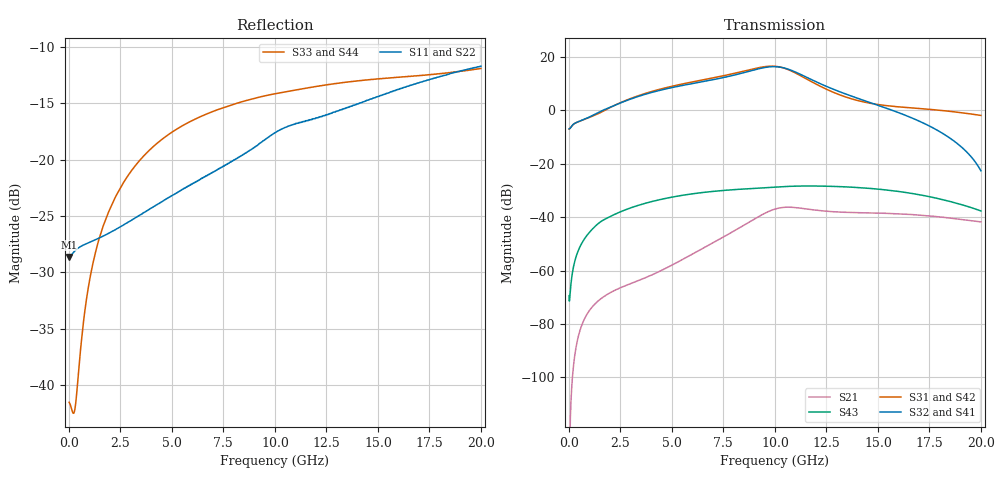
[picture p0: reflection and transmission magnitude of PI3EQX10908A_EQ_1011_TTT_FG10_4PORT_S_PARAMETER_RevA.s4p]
! NPort=4 DATA=2000 NOISE=0 GROUPDELAY=0 COMPLEX_DATAFORMAT=POLAR
! NumOfBlock=1 NumOfParam=0
! .MODEL Smodel S TSTONEFILE=PI3EQX10908A_EQ_1011_TTT_FG10_4PORT_S_PARAMETER_RevA.s4p TYPE=S
!  -- The above .MODEL line can be used for the S element in the netlist.
! The s parameter is extracted from the linear redriver, it is not bi-directional; only s(4,1)s(4,2) and s(3,1)s(3,2)
! should be the insertion loss
!Port definition:
!Port1 = input+
!Port2 = input-
!Port3 = output+
!Port4 = output-
# Hz S MA R  50
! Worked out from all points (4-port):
!   2000 points, 10 MHz to 20 GHz, reference 50 ohm
!   strongest paths, dB at 10 MHz, 5.01 GHz, 10.01 GHz, 15.01 GHz, 20 GHz:
!     S32: -6.9, 8.6, 16.4, 1.9, -22.6
!     S41: -6.9, 8.6, 16.4, 1.9, -22.5
!     S31: -6.9, 9.1, 16.5, 2.2, -1.9
!     S42: -6.9, 9.1, 16.5, 2.2, -1.8
!     S43: -69.4, -32.4, -28.7, -29.5, -37.6
!     S21: -127.2, -57.9, -36.9, -38.4, -41.7
!   lowest |S11| = -28.6 dB at 10 MHz (marker M1), VSWR 1.08, Z = 46.4 - j0.024 ohm
!   |S11| at or under -10 dB: start of sweep to end of sweep
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1e7  0.03701 -179.6  4.341e-07 14.6  0 0.0  0 0.0
     4.341e-07 14.6  0.03701 -179.6  0 0.0  0 0.0
     0.4507 1.1  0.4507 -178.9  0.008374 26.0  0.00034 -27.1
     0.4507 -178.9  0.4507 1.1  0.00034 -27.1  0.008374 26.0
6.73e9  0.08543 -120.0  0.002924 134.3  4.028e-07 64.3  2.109e-07 137.2
        0.002923 134.4  0.08545 -120.0  2.109e-07 137.2  4.029e-07 64.3
        3.89 -50.5  3.601 123.2  0.1601 12.0  0.02979 16.5
        3.601 123.2  3.89 -50.4  0.02979 16.5  0.1601 12.0
9.12e9  0.1153 -111.7  0.009843 110.9  2.515e-06 19.2  1.581e-06 115.4
        0.009847 111.0  0.1153 -111.7  1.582e-06 115.4  2.516e-06 19.2
        6.213 -111.4  5.905 63.1  0.1883 -6.6  0.03492 -8.1
        5.906 63.1  6.214 -111.4  0.03492 -8.1  0.1883 -6.6
1.033e10  0.1369 -112.1  0.01518 73.2  4.207e-06 -15.2  4.483e-06 81.0
          0.01518 73.2  0.1369 -112.1  4.485e-06 81.0  4.208e-06 -15.2
          6.39 -164.5  6.402 9.0  0.1987 -14.9  0.03731 -20.5
          6.403 9.1  6.39 -164.5  0.03731 -20.5  0.1987 -14.9
1.143e10  0.1479 -113.4  0.0145 41.9  5.008e-06 -25.1  7.639e-06 44.3
          0.01449 41.9  0.148 -113.4  7.643e-06 44.3  5.007e-06 -25.2
          4.094 154.4  4.382 -35.5  0.207 -21.1  0.03849 -33.7
          4.381 -35.5  4.094 154.4  0.03849 -33.7  0.207 -21.1
1.361e10  0.172 -111.8  0.01233 14.4  1.367e-05 -36.3  1.65e-05 -5.3
          0.01231 14.5  0.172 -111.8  1.65e-05 -5.3  1.367e-05 -36.3
          1.701 124.7  1.922 -83.1  0.2216 -32.5  0.0368 -60.1
          1.921 -83.1  1.701 124.7  0.0368 -60.1  0.2216 -32.5
2e10  0.26 -114.8  0.00821 -40.0  8.901e-05 -147.9  7.204e-05 -138.9
      0.008202 -39.7  0.2602 -114.8  7.206e-05 -138.9  8.899e-05 -147.9
      0.8073 54.3  0.07422 170.5  0.2539 -52.2  0.01317 -136.6
      0.07483 171.3  0.8085 54.3  0.01317 -136.6  0.2539 -52.2
